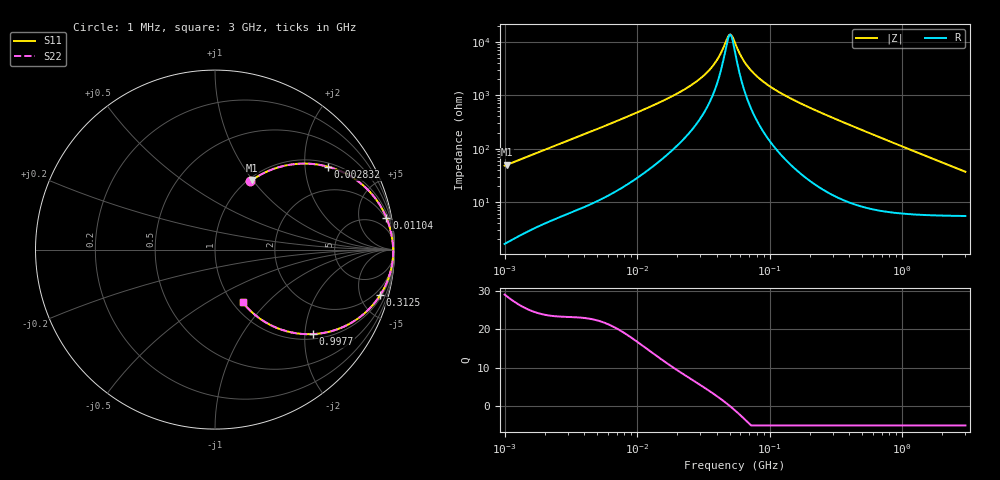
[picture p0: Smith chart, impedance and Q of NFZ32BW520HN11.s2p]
! NFZ32BW520HN11
# Hz S RI R 50
!Freq.(Hz) S11(Real) S11(Imag) S21(Real) S21(Imag) S12(Real) S12(Imag) S22(Real) S22(Imag)
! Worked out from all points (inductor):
!   401 points, 1 MHz to 3 GHz, reference 50 ohm
!   read as one part in series: L = 7.58 uH near 1.041 MHz
!   highest Q = 28.6 at 1.041 MHz (marker M1), where L = 7.63 uH
!   self-resonance near 49.56 MHz
!   S11 on the Smith chart (normalised r, x): 1 MHz: 1.03, +0.96; 2.832 MHz: 1.11, +2.64; 11.04 MHz: 2, +11; 312.5 MHz: 1.26, -7.21; 997.7 MHz: 1.12, -2.20; 3 GHz: 1.11, -0.73
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1000000  0.1953 0.3796  0.8047 -0.3796  0.8047 -0.3796  0.1953 0.3796
1040844  0.2075 0.3884  0.7925 -0.3884  0.7925 -0.3884  0.2075 0.3884
1786863  0.4198 0.4733  0.5802 -0.4733  0.5802 -0.4733  0.4198 0.4733
2831560  0.6311 0.4615  0.3689 -0.4615  0.3689 -0.4615  0.6311 0.4615
3823119  0.7506 0.4115  0.2494 -0.4115  0.2494 -0.4115  0.7506 0.4115
1.104425e7  0.9549 0.1781  0.0451 -0.1781  0.0451 -0.1781  0.9549 0.1781
1.461624e7  0.9712 0.1323  0.0288 -0.1323  0.0288 -0.1323  0.9712 0.1323
2.362996e7  0.9855 0.0714  0.0145 -0.0714  0.0145 -0.0714  0.9855 0.0714
3.254976e7  0.9901 0.0392  0.00995 -0.0392  0.00995 -0.0392  0.9901 0.0392
3.976269e7  0.9917 0.0209  0.00828 -0.0209  0.00828 -0.0209  0.9917 0.0209
4.955604e7  0.9927 0.00129  0.0073 -0.00129  0.0073 -0.00129  0.9927 0.00129
5.15801e7  0.9928 -0.00226  0.00722 0.00226  0.00722 0.00226  0.9928 -0.00226
5.477226e7  0.9929 -0.00762  0.00714 0.00762  0.00714 0.00762  0.9929 -0.00762
6.558369e7  0.9927 -0.024  0.00735 0.024  0.00735 0.024  0.9927 -0.024
8.338914e7  0.9913 -0.0472  0.00874 0.0472  0.00874 0.0472  0.9913 -0.0472
1.219755e8  0.9854 -0.09  0.0146 0.09  0.0146 0.09  0.9854 -0.09
2.094008e8  0.962 -0.1715  0.038 0.1715  0.038 0.1715  0.962 -0.1715
3.124888e8  0.9209 -0.2528  0.0791 0.2528  0.0791 0.2528  0.9209 -0.2528
8.005644e8  0.6479 -0.4546  0.3521 0.4546  0.3521 0.4546  0.6479 -0.4546
9.977393e8  0.5464 -0.4709  0.4536 0.4709  0.4536 0.4709  0.5464 -0.4709
1.818868e9  0.2861 -0.4077  0.7139 0.4077  0.7139 0.4077  0.2861 -0.4077
3e9  0.1537 -0.2932  0.8463 0.2932  0.8463 0.2932  0.1537 -0.2932
